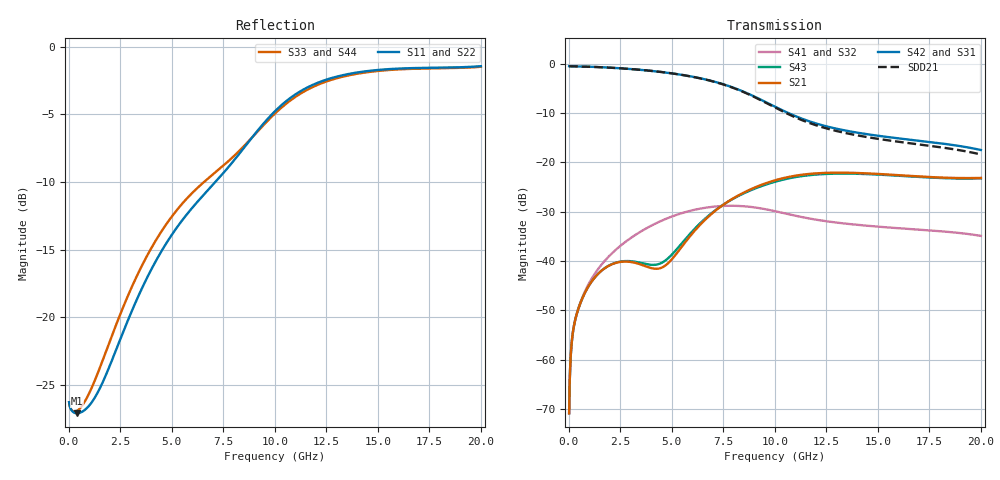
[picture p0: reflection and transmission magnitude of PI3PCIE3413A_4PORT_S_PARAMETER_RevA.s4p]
! NPort=4 DATA=800 NOISE=0 GROUPDELAY=0 COMPLEX_DATAFORMAT=POLAR
! NumOfBlock=1 NumOfParam=0
! .MODEL Smodel S TSTONEFILE=PI3PCIE3413A_4PORT_S_PARAMETER_RevA.s4p TYPE=S
!  -- The above .MODEL line can be used for the S element in the netlist.
!PORT1 = INPUT+
!PORT2 = INPUT-
!PORT3 = OUTPUT+
!PORT4 = OUTPUT-
# Hz S MA R  50
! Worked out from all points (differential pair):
!   800 points, 25 MHz to 20 GHz, reference 50 ohm
!   strongest paths, dB at 25 MHz, 5.025 GHz, 10.03 GHz, 15.03 GHz, 20 GHz:
!     S42: -0.5, -1.9, -8.7, -14.6, -17.5
!     S31: -0.5, -1.9, -8.7, -14.6, -17.5
!     S21: -70.9, -39.6, -23.6, -22.3, -23.1
!     S43: -70.9, -38.6, -23.9, -22.5, -23.2
!     S41: -70.9, -31.0, -29.9, -33.0, -34.9
!     S32: -70.9, -31.0, -29.9, -33.0, -34.9
!   taken as a pair (ports 2,1 in; 4,3 out), SDD21 dB: -0.5, -1.9, -8.9, -15.2, -18.4
!   lowest |S11| = -27.1 dB at 400 MHz (marker M1), VSWR 1.09, Z = 54.6 + j0.311 ohm
!   |S11| at or under -10 dB: start of sweep to 7.119 GHz
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2.5e7  0.04846 -2.5  0.0002853 86.0  0.9475 -0.6  0.0002846 86.0
       0.0002853 86.0  0.04846 -2.5  0.0002846 86.0  0.9475 -0.6
       0.9475 -0.6  0.0002846 86.0  0.0485 -2.3  0.0002853 86.1
       0.0002846 86.0  0.9475 -0.6  0.0002853 86.1  0.0485 -2.3
4e8  0.04411 3.7  0.002921 64.3  0.9418 -7.4  0.002938 63.9
     0.002921 64.3  0.04411 3.7  0.002938 63.9  0.9418 -7.4
     0.9418 -7.4  0.002938 63.9  0.04501 7.8  0.00292 64.5
     0.002938 63.9  0.9418 -7.4  0.00292 64.5  0.04501 7.8
1.85e9  0.06215 24.8  0.008701 55.5  0.9193 -33.6  0.01056 51.7
        0.008701 55.5  0.06215 24.8  0.01056 51.7  0.9193 -33.6
        0.9192 -33.6  0.01056 51.7  0.07592 29.5  0.008721 56.5
        0.01056 51.7  0.9192 -33.6  0.008721 56.5  0.07592 29.5
4.05e9  0.1521 15.6  0.008427 60.2  0.8473 -73.4  0.02305 16.1
        0.008427 60.2  0.1521 15.6  0.02305 16.1  0.8473 -73.4
        0.8471 -73.4  0.02304 16.0  0.1822 13.4  0.009129 63.1
        0.02304 16.0  0.8471 -73.4  0.009129 63.1  0.1822 13.4
7.675e9  0.3533 -17.9  0.03934 92.0  0.605 -141.6  0.03628 -58.1
         0.03934 92.0  0.3533 -17.9  0.03628 -58.1  0.605 -141.6
         0.6048 -141.7  0.03627 -58.2  0.3732 -24.6  0.03925 88.1
         0.03627 -58.2  0.6048 -141.7  0.03925 88.1  0.3732 -24.6
1.35e10  0.7914 -74.8  0.0786 25.5  0.2094 156.2  0.02387 -146.7
         0.0786 25.5  0.7914 -74.8  0.02387 -146.7  0.2094 156.2
         0.2092 156.1  0.02385 -146.8  0.7819 -75.6  0.07698 25.4
         0.02385 -146.8  0.2092 156.1  0.07698 25.4  0.7819 -75.6
2e10  0.8483 -106.6  0.06959 -3.9  0.1338 87.1  0.01799 127.1
      0.06959 -3.9  0.8483 -106.6  0.01799 127.1  0.1338 87.1
      0.1337 86.9  0.01797 126.9  0.8438 -106.8  0.06892 -3.6
      0.01797 126.9  0.1337 86.9  0.06892 -3.6  0.8438 -106.8
